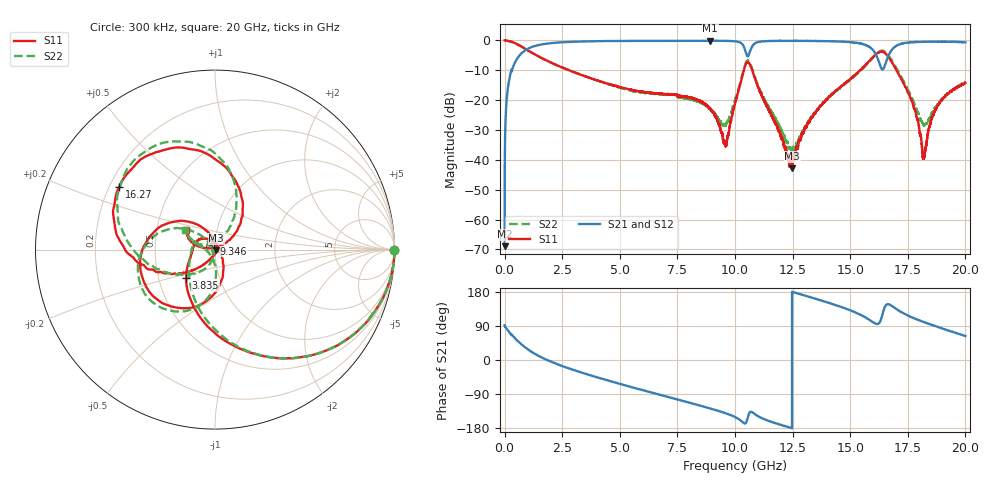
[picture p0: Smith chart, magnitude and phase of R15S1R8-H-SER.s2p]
!{R15S1R8}
!Johanson Technology Inc.
!www.johansontechnology.com
!Test Board Conditions:
!Substrate Type  RO4350B
!Substrate Thickness  20 mil
!Substrate Dk  3.66
!TL Type: GCPW
!TL Trace Width  34 mil
!TL Gap  10 mil
!Electrode orientation  Horizontal
!DUT TOPOLOGY	SERIES
!Mounting Pad LxW  26x52 mil
! Created Sat Feb  6 12:18:17 2021
# hz S ma R 50
! 2 Port Network Data from SP1.SP block
! freq  magS11  angS11  magS21  angS21  magS12  angS12  magS22  angS22
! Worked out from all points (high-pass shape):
!   20001 points, 300 kHz to 20 GHz, reference 50 ohm
!   highest |S21| = -0.10 dB at 8.925 GHz (marker M1); lowest = -68.9 dB at 300 kHz (marker M2)
!   |S21| within 3 dB of the highest: 934.4 MHz to 10.44 GHz (9.501 GHz wide, 167 % of centre); 10.68 GHz to 15.98 GHz (5.296 GHz wide, 39.7 % of centre)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
!   lowest |S11| = -42.9 dB at 12.48 GHz (marker M3), VSWR 1.01, Z = 50.7 - j0.303 ohm
!   |S11| at or under -10 dB: 2.795 GHz to 10.38 GHz (7.587 GHz wide, 115 % of centre); 10.75 GHz to 15.43 GHz (4.678 GHz wide, 35.7 % of centre); 17.01 GHz to end of sweep
!   |S22| runs from -38.0 to 0.0 dB; largest |S21 - S12| = 0.018
!   S11 on the Smith chart (normalised r, x): 300 kHz: open; 3.835 GHz: 0.69, -0.23; 9.346 GHz: 0.99, +0.07; 16.27 GHz: 0.24, +0.28; 20 GHz: 0.71, +0.16
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300000  0.9991 -0.2  0.0003595 91.6  0.0003331 71.1  0.9976 -0.1
1.313e8  0.9882 -10.7  0.1487 79.0  0.1496 79.0  0.9874 -10.7
4.833e8  0.8897 -34.2  0.4526 55.5  0.4534 55.6  0.8885 -34.3
1.6023e9  0.5092 -83.9  0.8559 6.8  0.8571 6.8  0.5087 -82.2
3.3343e9  0.2643 -126.2  0.9597 -33.0  0.9597 -33.1  0.2653 -118.9
3.8353e9  0.226 -135.2  0.9695 -42.5  0.9688 -42.4  0.2263 -128.4
6.6673e9  0.129 -174.8  0.9835 -90.6  0.9841 -90.6  0.1273 171.8
8.9253e9  0.07242 124.5  0.9886 -127.9  0.9875 -127.9  0.07009 169.3
9.3463e9  0.03498 99.2  0.986 -135.5  0.9869 -135.6  0.04463 -170.4
9.6183e9  0.01851 15.9  0.9829 -141.0  0.9823 -141.0  0.03978 -127.6
1.00003e10  0.08767 -59.3  0.9674 -150.3  0.9671 -150.3  0.09954 -88.9
1.06013e10  0.4253 -169.9  0.5784 -142.1  0.5792 -142.4  0.4471 -164.0
1.08643e10  0.2324 136.9  0.8941 -143.0  0.8942 -143.2  0.2438 150.6
1.24763e10  0.007186 -24.6  0.9838 180.0  0.9849 -180.0  0.01327 -167.4
1.33343e10  0.05092 -112.3  0.9801 164.5  0.9813 164.6  0.05331 -104.6
1.54903e10  0.3297 -157.8  0.8798 117.9  0.8847 118.0  0.3245 -159.6
1.62673e10  0.6378 146.7  0.4165 98.2  0.4141 98.5  0.6505 141.8
1.66673e10  0.5245 93.0  0.5664 147.1  0.5599 148.3  0.562 93.7
1.77383e10  0.08069 32.8  0.9352 111.1  0.9368 110.6  0.09577 57.3
1.82013e10  0.01118 98.7  0.9482 100.2  0.9545 100.1  0.03831 103.2
1.87603e10  0.07648 170.4  0.9519 88.1  0.953 88.2  0.08185 160.1
2e10  0.1936 145.7  0.9275 63.2  0.9224 63.0  0.2027 146.5
